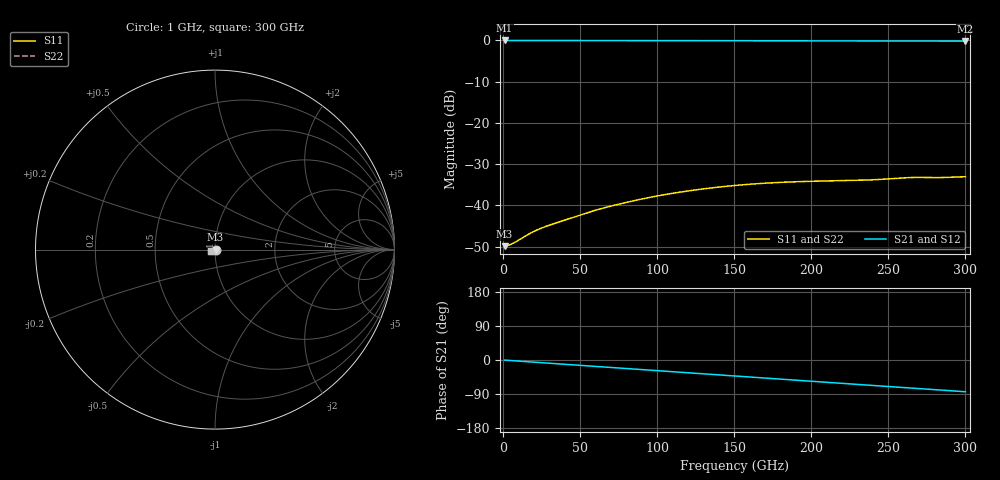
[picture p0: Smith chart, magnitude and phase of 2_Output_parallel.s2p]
#  Hz  S  RI  R  50
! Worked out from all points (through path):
!   300 points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, 1 GHz to 300 GHz, reference 50 ohm
!   highest |S21| = -0.03 dB at 1 GHz (marker M1); lowest = -0.2 dB at 300 GHz (marker M2)
!   group delay of S21, straight-line fit = 776 fs
!   lowest |S11| = -49.9 dB at 1 GHz (marker M3), VSWR 1.01, Z = 50.3 + j0.00178 ohm
!   |S11| at or under -10 dB: start of sweep to end of sweep
!   |S22| runs from -49.9 to -33.0 dB; largest |S21 - S12| = 0.0002
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1e9  0.0032 1.77e-05  0.9969 -0.00507  0.9969 -0.00507  0.0032 1.93e-05
3e9  0.00326 4.58e-05  0.9967 -0.0152  0.9967 -0.0152  0.00325 5.05e-05
6e9  0.00343 4.53e-05  0.9961 -0.0303  0.9961 -0.0303  0.00343 5.31e-05
1.7e10  0.00446 -0.000751  0.9917 -0.0845  0.9917 -0.0844  0.00446 -0.000752
2.4e10  0.0049 -0.00179  0.9877 -0.1182  0.9877 -0.1182  0.0049 -0.0018
3.1e10  0.00506 -0.00292  0.9828 -0.152  0.9828 -0.152  0.00505 -0.00292
5.1e10  0.00486 -0.00604  0.9621 -0.2468  0.9621 -0.2468  0.00486 -0.00605
6.1e10  0.00439 -0.00768  0.9486 -0.2932  0.9486 -0.2932  0.00439 -0.00768
7.2e10  0.0036 -0.00935  0.931 -0.3435  0.931 -0.3435  0.0036 -0.00934
8.7e10  0.00221 -0.0114  0.9029 -0.4102  0.9029 -0.4102  0.00221 -0.0114
1.01e11  0.000569 -0.0131  0.8724 -0.4706  0.8724 -0.4706  0.000567 -0.0131
1.13e11  -0.00103 -0.0143  0.843 -0.5205  0.843 -0.5205  -0.00102 -0.0143
1.26e11  -0.00288 -0.0152  0.8081 -0.5725  0.8081 -0.5725  -0.00289 -0.0152
1.51e11  -0.00662 -0.0162  0.7319 -0.6659  0.7319 -0.6659  -0.00662 -0.0162
1.74e11  -0.00985 -0.016  0.6521 -0.7431  0.6521 -0.7431  -0.00985 -0.016
2.01e11  -0.0128 -0.0148  0.5477 -0.8214  0.5477 -0.8214  -0.0128 -0.0148
2.18e11  -0.0142 -0.014  0.4769 -0.8628  0.477 -0.8628  -0.0142 -0.014
2.35e11  -0.0152 -0.0133  0.403 -0.8978  0.403 -0.8978  -0.0152 -0.0133
2.51e11  -0.0165 -0.013  0.3319 -0.9243  0.3319 -0.9243  -0.0165 -0.013
2.64e11  -0.018 -0.0122  0.2735 -0.9424  0.2734 -0.9424  -0.018 -0.0122
2.84e11  -0.0192 -0.0103  0.1811 -0.963  0.1812 -0.963  -0.0192 -0.0103
3e11  -0.0205 -0.00877  0.1066 -0.9734  0.1065 -0.9733  -0.0205 -0.00875
